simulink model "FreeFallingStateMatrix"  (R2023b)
settings: Solver=VariableStepAuto  StartTime=0.0  StopTime=10.0  MaxStep=.001  RelTol=1e-3

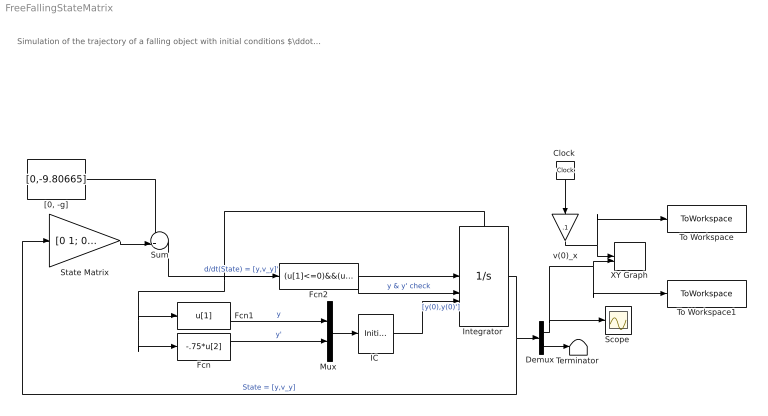
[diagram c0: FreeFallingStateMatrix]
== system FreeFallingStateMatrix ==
  note: Simulation of the trajectory of a falling object with initial conditions $\ddot{y}=-g$ $\ddot{x}=0$ $\dot{y}(0)=v_{y}(0)$ $\dot{x}=v_x(0)$ $y(0)=y_0$ $x(0)=x_0$
  "Clock " : Clock
  "Demux " : Demux  Outputs=2
  Fcn : Fcn  Expr=-.75*u[2]
  Fcn1 : Fcn  Expr=u[1]
  Fcn2 : Fcn  Expr=(u[1]<=0)&&(u[2]<0)
  "IC " : InitialCondition  Value=[10, 5]
  "Integrator " : Integrator  ExternalReset=rising  InitialConditionSource=external  LowerSaturationLimit=0  ShowStatePort=on
  "Mux " : Mux  Inputs=2
  "Scope " : Scope
  State Matrix : Gain  Gain=[0 1; 0 0]  Multiplication=Matrix(K*u)
  Sum : Sum  Inputs=++|
  "Terminator " : Terminator
  To Workspace : ToWorkspace  VariableName=x_pos  SaveFormat=Timeseries  SampleTime=-1
  To Workspace1 : ToWorkspace  VariableName=y_pos  SaveFormat=Timeseries  SampleTime=-1
  XY Graph : Record  FileSettingsInternal="{\"entries\":[{\"content\":{\"excelSettings\":{\"content\":{},\"type\":\"Streamout.ExcelSettings\"}},\"type\":\"Streamout.FileSettingStorage\",\"uuid\":\"\"}],\"packageUris\":[\"http:\\/\\/schema.mathworks.com\\/mf0\\/streamout_blocks\\/R2020a\"],\"version\":\"1.0\"}"  Layout=[1 1]  SignalsInternal="{\"entries\":[{\"content\":{\"signals\":[{\"content\":{\"blockPath\":[],\"dimensions\":[1],\"domain\":\"\",\"lineColor\":\"#4dbeee\",\"plots\":[ 1 ],\"port\":1,\"signalID\":1,\"signalName\":\"v(0)_x\"},\"type\":\"RecordBlkView.Signal\",\"uuid\":\"\"},{\"content\":{\"blockPath\":[],\"dimensions\":[1],\"domain\":\"\",\"lineColor\":\"#a2142f\",\"plots\":[ 1 ],\"port\":2,\"signalID\":2,\"signalName\":\"Demux :1\"},\"type\":\"RecordBlkView.Signal\",\"uuid\":\"\"}]},\"type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"  VisualizationBindings="{\"xyplotplugin\":{\"info\":[{\"series\":[{\"bindingParametersList\":[{\"parameter\":\"X-Axis\",\"signalID\":1,\"signalName\":\"v(0)_x\"},{\"parameter\":\"Y-Axis\",\"signalID\":2,\"signalName\":\"Demux :1\"}],\"seriesID\":0}],\"subplotID\":1}]}}"  CompatibilityTag=XY
  "[0, -g]" : Constant  Value=[0,-9.80665]
  v(0)_x : Gain  Gain=.1
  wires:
  "[0, -g]"/1 -> Sum/1
  State Matrix/1 -> Sum/2
  Sum/1 -> "Integrator "/1  "d/dt(State) = [y,v_y]'"
  "Integrator "/1 -> "Demux "/1, State Matrix/1  "State = [y,v_y]"
  "Demux "/1 -> "Scope "/1, To Workspace1/1, XY Graph/2
  "IC "/1 -> "Integrator "/3  "[y(0),y(0)']"
  Fcn2/1 -> "Integrator "/2  "y & y' check"
  Fcn1/1 -> "Mux "/1  "y"
  Fcn/1 -> "Mux "/2  "y'"
  "Mux "/1 -> "IC "/1
  "Integrator "/State -> Fcn/1, Fcn1/1, Fcn2/1
  "Clock "/1 -> v(0)_x/1
  v(0)_x/1 -> To Workspace/1, XY Graph/1
  "Demux "/2 -> "Terminator "/1
